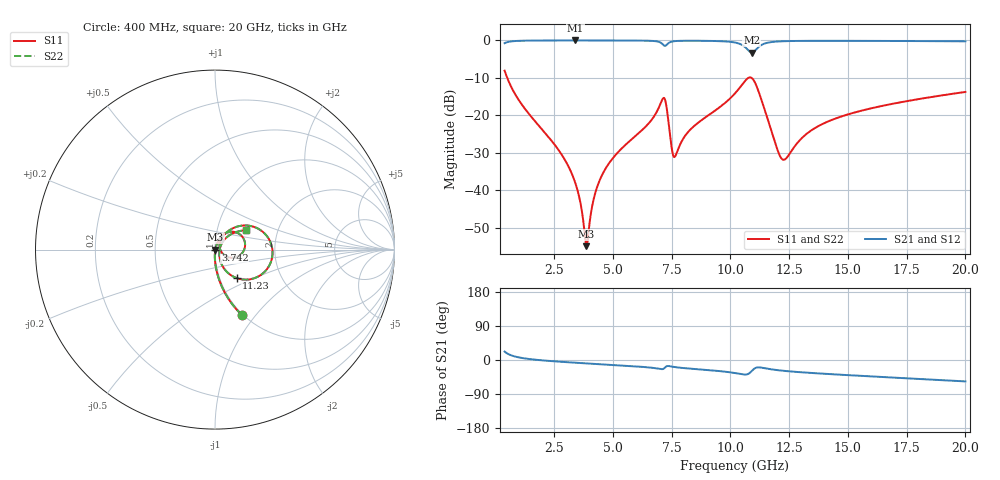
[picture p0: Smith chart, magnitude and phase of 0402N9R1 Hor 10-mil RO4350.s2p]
# GHz S MA R 50
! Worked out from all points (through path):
!   1960 points, 400 MHz to 20 GHz, reference 50 ohm
!   highest |S21| = -0.02 dB at 3.402 GHz (marker M1); lowest = -3.2 dB at 10.92 GHz (marker M2)
!   group delay of S21, straight-line fit = 8.34 ps
!   lowest |S11| = -54.8 dB at 3.882 GHz (marker M3), VSWR 1.00, Z = 50.2 - j0.0359 ohm
!   |S11| at or under -10 dB: 512 MHz to 10.77 GHz (10.25 GHz wide, 182 % of centre); 10.91 GHz to end of sweep
!   |S22| runs from -54.8 to -8.1 dB; largest |S21 - S12| = 0
!   S11 on the Smith chart (normalised r, x): 400 MHz: 0.99, -0.85; 3.742 GHz: 1.00, -0.01; 11.23 GHz: 1.20, -0.40; 20 GHz: 1.38, +0.31
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0.4  0.3946 -67.6  0.9183 22.3  0.9183 22.3  0.3946 -67.6
1.280449  0.1208 -85.6  0.9916 4.0  0.9916 4.0  0.1208 -85.6
2.7512  0.03264 -91.9  0.9979 -4.5  0.9979 -4.5  0.03264 -91.9
3.401531  0.01274 -89.7  0.9981 -7.2  0.9981 -7.2  0.01274 -89.7
3.671669  0.00569 -80.4  0.9981 -8.2  0.9981 -8.2  0.00569 -80.4
3.741705  0.004021 -72.5  0.9981 -8.5  0.9981 -8.5  0.004021 -72.5
3.881776  0.00181 -11.4  0.998 -9.0  0.998 -9.0  0.00181 -11.4
4.22195  0.008457 66.5  0.9979 -10.3  0.9979 -10.3  0.008457 66.5
4.622154  0.01786 71.5  0.9975 -11.7  0.9975 -11.7  0.01786 71.5
6.943338  0.124 52.0  0.9603 -22.9  0.9603 -22.9  0.124 52.0
7.223481  0.1624 -0.3  0.8452 -19.8  0.8452 -19.8  0.1624 -0.3
7.513629  0.03568 -17.1  0.964 -17.3  0.964 -17.3  0.03568 -17.1
7.633691  0.02798 19.1  0.9774 -18.6  0.9774 -18.6  0.02798 19.1
8.294028  0.06447 59.9  0.9893 -22.8  0.9893 -22.8  0.06447 59.9
10.205  0.1975 42.3  0.936 -34.5  0.936 -34.5  0.1975 42.3
10.60521  0.2823 21.0  0.826 -38.4  0.826 -38.4  0.2823 21.0
10.91536  0.3151 -16.5  0.6895 -28.9  0.6895 -28.9  0.3151 -16.5
11.22552  0.199 -52.8  0.8274 -19.4  0.8274 -19.4  0.199 -52.8
12.21603  0.02597 -17.1  0.974 -28.2  0.974 -28.2  0.02597 -17.1
13.46667  0.06386 45.7  0.9863 -34.3  0.9863 -34.3  0.06386 45.7
16.73834  0.1396 41.6  0.9831 -45.8  0.9831 -45.8  0.1396 41.6
20  0.2056 31.9  0.9719 -56.5  0.9719 -56.5  0.2056 31.9
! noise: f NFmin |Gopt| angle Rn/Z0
0.4  0.001221  0.78  1.696  0.001137
2.571  0.004981  0.6736  6.147  0.002932
4.752  0.008413  0.6493  10.9  0.004516
6.933  0.03793  0.8719  15.95  0.06259
9.104  0.02424  0.755  20.72  0.01935
11.29  0.1088  0.9264  25.87  0.3114
13.47  0.03143  0.7297  30.49  0.02159
15.64  0.02698  0.6546  34.78  0.01361
17.82  0.02701  0.6204  38.96  0.01188
20  0.02821  0.6026  43.03  0.01144
